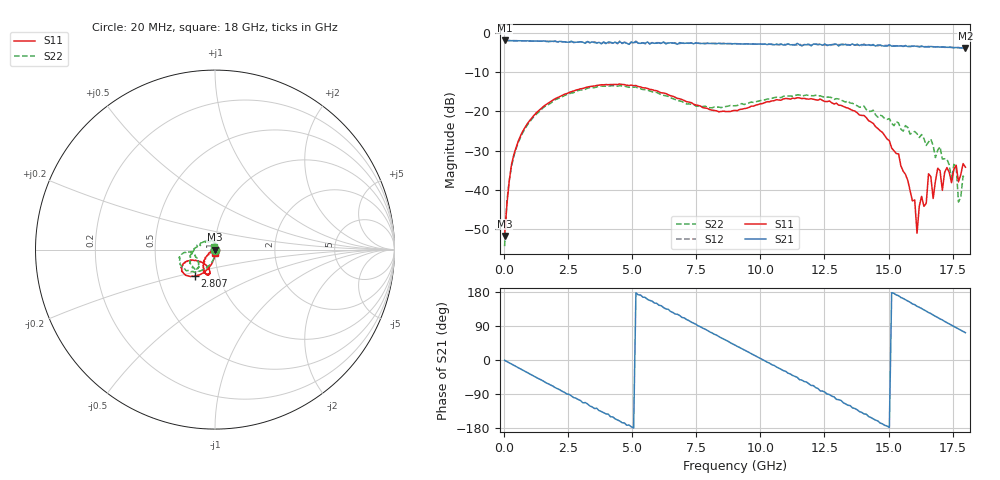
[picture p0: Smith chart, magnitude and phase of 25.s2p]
!Agilent Technologies,N5230A,US43500223,A.07.50.48
!Agilent N5230A: A.07.50.48
!Date: Sunday, January 17, 2016 15:26:44
!Correction: S11(Full 2 Port(1,2))
!S21(Full 2 Port(1,2))
!S12(Full 2 Port(1,2))
!S22(Full 2 Port(1,2))
!S2P File: Measurements: S11, S21, S12, S22:
# Hz S  dB  R 50
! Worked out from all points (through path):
!   201 points, 20 MHz to 18 GHz, reference 50 ohm
!   highest |S21| = -1.97 dB at 20 MHz (marker M1); lowest = -3.9 dB at 18 GHz (marker M2)
!   group delay of S21, straight-line fit = 99.5 ps
!   lowest |S11| = -51.7 dB at 20 MHz (marker M3), VSWR 1.01, Z = 49.8 - j0.0955 ohm
!   |S11| at or under -10 dB: start of sweep to end of sweep
!   |S22| runs from -54.4 to -13.5 dB; largest |S21 - S12| = 0.044
!   S11 on the Smith chart (normalised r, x): 20 MHz: 1.00, -0.00; 2.807 GHz: 0.77, -0.24; 18 GHz: 1.00, -0.04
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2e7  -51.73 -158.3  -1.97 -0.8  -1.98 -0.9  -54.36 -153.9
1.998e8  -37.80 -90.0  -2.01 -7.5  -2.01 -7.5  -37.70 -87.8
6.493e8  -26.16 -95.8  -2.05 -23.9  -2.06 -24.0  -26.53 -96.9
2.8069e9  -14.62 -127.2  -2.42 -101.0  -2.36 -101.7  -14.97 -136.9
3.0766e9  -14.20 -130.8  -2.42 -113.1  -2.35 -111.9  -14.62 -140.4
4.515e9  -13.07 -146.7  -2.28 -161.1  -2.11 -160.5  -13.48 -161.0
6.0433e9  -15.06 -157.4  -2.58 144.5  -2.55 143.1  -15.50 -174.8
7.4817e9  -18.40 -148.5  -2.59 94.5  -2.64 93.2  -18.66 -164.2
9.01e9  -19.79 -117.9  -2.77 39.4  -2.82 39.0  -18.58 -139.9
1.04484e10  -17.37 -103.2  -2.97 -12.4  -2.96 -13.0  -16.72 -133.1
1.20666e10  -16.95 -113.6  -2.89 -67.5  -3.12 -69.8  -16.07 -150.4
1.32353e10  -18.75 -123.7  -3.09 -112.7  -2.90 -113.8  -17.42 -169.4
1.50333e10  -27.50 -149.7  -3.06 -178.1  -3.31 -179.0  -21.89 149.3
1.60222e10  -42.59 -130.8  -3.40 145.9  -3.48 143.9  -25.15 110.0
1.61121e10  -51.05 -106.7  -3.48 141.8  -3.44 140.9  -25.70 102.4
1.65616e10  -35.92 -35.0  -3.60 125.3  -3.51 124.2  -27.82 100.7
1.67414e10  -42.23 -42.7  -3.56 118.6  -3.60 117.5  -28.72 87.5
1.69212e10  -34.51 -36.0  -3.56 112.1  -3.64 110.5  -29.88 99.8
1.7101e10  -40.15 -59.4  -3.60 105.7  -3.67 104.1  -32.19 80.4
1.76404e10  -33.73 -66.9  -3.77 85.4  -3.83 83.8  -34.07 100.0
1.77303e10  -37.97 -76.0  -3.78 81.8  -3.79 80.4  -43.11 109.3
1.8e10  -34.24 -83.4  -3.89 72.1  -3.92 70.2  -37.19 104.8
